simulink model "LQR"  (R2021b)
settings: Solver=VariableStepAuto  StartTime=0.0  StopTime=10.0  RelTol=1e-3
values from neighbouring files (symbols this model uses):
  Ts = 0.01    [CompareGazeboSimulink.m]    (also in RobotModel.m = 0.05)
libraries: cstblocks x1

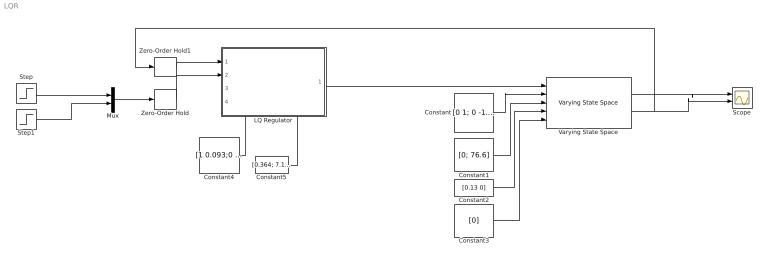
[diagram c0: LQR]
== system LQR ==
  Constant : Constant  Value=[0 1; 0 -1.53]
  Constant1 : Constant  Value=[0; 76.6]  VectorParams1D=off
  Constant2 : Constant  Value=[0.13 0]  VectorParams1D=off
  Constant3 : Constant  Value=[0]  VectorParams1D=off
  Constant4 : Constant  Value=[1 0.093;0 0.858]  VectorParams1D=off
  Constant5 : Constant  Value=[0.364; 7.112]  VectorParams1D=off
  LQ Regulator : Subsystem
  Mux : Mux  Inputs=2
  Scope : Scope  NumInputPorts=2
  Step : Step  After=55  SampleTime=0
  Step1 : Step  After=0  SampleTime=0
  Varying State Space : cstblocks/Linear Parameter Varying/Varying State Space  x0=[10; 20]  xNames=''  OutputX=on  OutputDX=off
  Zero-Order Hold : ZeroOrderHold  SampleTime=Ts
  Zero-Order Hold1 : ZeroOrderHold  SampleTime=Ts
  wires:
  Constant/1 -> Varying State Space/2
  Constant1/1 -> Varying State Space/3
  Constant2/1 -> Varying State Space/4
  Constant3/1 -> Varying State Space/5
  Varying State Space/1 -> Scope/1
  Varying State Space/2 -> Zero-Order Hold1/1, Scope/2
  Mux/1 -> Zero-Order Hold/1
  Zero-Order Hold/1 -> LQ Regulator/2(Desired State)
  Zero-Order Hold1/1 -> LQ Regulator/1(Actual State)
  Step/1 -> Mux/1
  Step1/1 -> Mux/2
  LQ Regulator/1(Output) -> Varying State Space/1
  Constant4/1 -> LQ Regulator/3(A)
  Constant5/1 -> LQ Regulator/4(B)

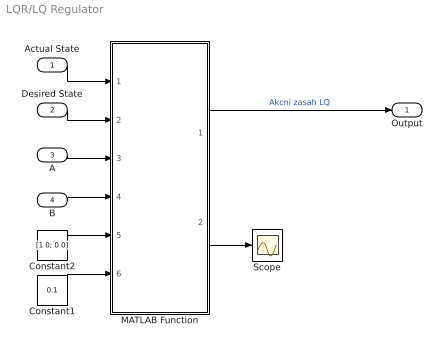
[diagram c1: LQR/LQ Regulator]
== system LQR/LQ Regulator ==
  Actual State : Inport
  Desired State : Inport  Port=2
  A : Inport  Port=3
  B : Inport  Port=4
  Constant1 : Constant  Value=0.1
  Constant2 : Constant  Value=[1 0; 0 0]  VectorParams1D=off
  MATLAB Function : MATLAB Function  TreatAsAtomicUnit=on
  Scope : Scope
  Output : Outport
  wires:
  MATLAB Function/2(K) -> Scope/1
  Constant1/1 -> MATLAB Function/6(R)
  Constant2/1 -> MATLAB Function/5(Q)
  B/1 -> MATLAB Function/4(B)
  A/1 -> MATLAB Function/3(A)
  Desired State/1 -> MATLAB Function/2(DesiredState)
  Actual State/1 -> MATLAB Function/1(ActualState)
  MATLAB Function/1(u) -> Output/1  "Akcní zasah LQ"

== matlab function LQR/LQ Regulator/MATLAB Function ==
function [u, K]   = lq(ActualState, DesiredState, A, B, Q, R)                                                     

K_old = [0 0];
K     = [1 1];

P = Q;

while (K ~= K_old)
    K_old = K;
    P = Q + K'*R*K + (A - B*K)'*P*(A - B*K);
    K = (R + B'*P*B)^(-1)*B'*P*A;
end

u = -K*(ActualState - DesiredState);
end
